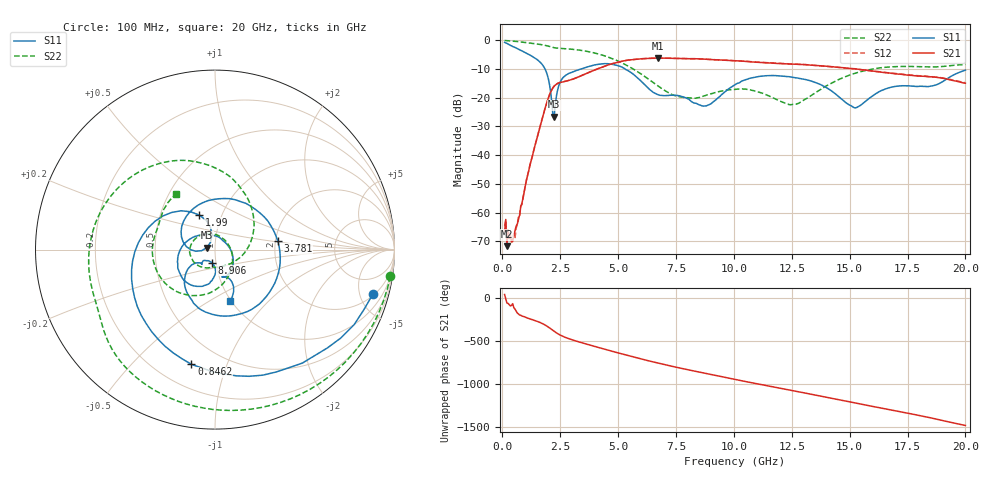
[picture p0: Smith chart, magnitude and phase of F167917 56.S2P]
!  2-Port S-parameters saved by WinCal
! VAR MeasName=S-Parameters (CALIBRATED_DATA) read from VNA (N5242A)
! VAR MeasDate=2016-11-22 9:02:42
! VAR NAME=F167917 56
! VAR FILENAME=F167917 56.S2P
! VAR DATE=2016-11-22 9:02:42
! VAR PHYS_PORTS=1,2
# Hz S DB R 50
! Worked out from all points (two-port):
!   401 points, 100 MHz to 20 GHz, reference 50 ohm
!   highest |S21| = -6.24 dB at 6.717 GHz (marker M1); lowest = -71.7 dB at 199.5 MHz (marker M2)
!   |S21| within 3 dB of the highest: 4.368 GHz to 14.27 GHz (9.899 GHz wide, 106 % of centre)
!   lowest |S11| = -26.7 dB at 2.239 GHz (marker M3), VSWR 1.10, Z = 45.7 + j0.997 ohm
!   |S11| at or under -10 dB: 1.843 GHz to 3.416 GHz (1.573 GHz wide, 59.8 % of centre); 5.297 GHz to end of sweep
!   |S22| runs from -22.5 to -0.1 dB; largest |S21 - S12| = 0.0045
!   S11 on the Smith chart (normalised r, x): 100 MHz: 2.18, -6.58; 846.2 MHz: 0.34, -0.76; 1.99 GHz: 0.78, +0.32; 3.781 GHz: 2.06, +0.23; 8.906 GHz: 0.95, -0.14; 20 GHz: 0.99, -0.63
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1e8  -0.78 -15.6  -66.37 43.0  -64.71 44.9  -0.10 -8.7
1.995e8  -1.10 -28.5  -71.66 -55.5  -69.63 -56.4  -0.16 -16.9
4.98e8  -2.36 -63.4  -67.62 -109.2  -67.31 -105.4  -0.36 -40.7
8.4625e8  -3.70 -101.6  -56.71 153.3  -57.18 155.5  -0.67 -66.9
1.44325e9  -6.41 -166.3  -35.73 97.7  -35.73 97.9  -1.27 -106.8
1.9905e9  -13.48 114.5  -20.07 24.6  -20.06 24.7  -2.08 -138.9
2.23925e9  -26.65 166.4  -16.02 -24.4  -16.00 -24.2  -2.61 -150.4
2.5875e9  -13.39 151.9  -14.56 -79.5  -14.53 -79.5  -2.89 -164.8
3.43325e9  -9.96 44.7  -12.30 -157.4  -12.29 -157.4  -3.59 157.1
3.7815e9  -9.05 7.9  -11.08 175.7  -11.07 175.9  -4.09 141.2
5.1745e9  -9.39 -105.6  -7.32 72.1  -7.29 72.1  -7.95 74.7
6.71675e9  -18.94 -139.4  -6.24 -33.5  -6.24 -33.5  -15.88 -8.9
6.7665e9  -19.07 -138.5  -6.24 -36.6  -6.24 -36.7  -16.17 -11.9
7.7615e9  -19.61 -134.4  -6.39 -96.7  -6.39 -96.7  -19.84 -69.3
8.90575e9  -22.55 -104.6  -6.68 -162.1  -6.68 -162.1  -18.89 -116.1
1.005e10  -15.55 -94.7  -7.15 135.9  -7.14 136.0  -17.15 -161.5
1.204e10  -12.48 -144.4  -8.15 32.0  -8.09 31.7  -21.37 91.3
1.338325e10  -14.33 179.3  -8.69 -38.8  -8.69 -39.0  -19.06 -28.9
1.5224e10  -23.53 50.5  -9.94 -136.6  -10.01 -136.7  -11.55 -106.7
1.67165e10  -16.54 -54.3  -11.41 145.0  -11.43 145.5  -9.33 -154.0
1.805975e10  -16.02 -75.0  -12.48 74.2  -12.40 74.5  -9.23 170.7
2e10  -10.43 -73.8  -14.97 -39.1  -14.83 -39.0  -8.47 124.8
